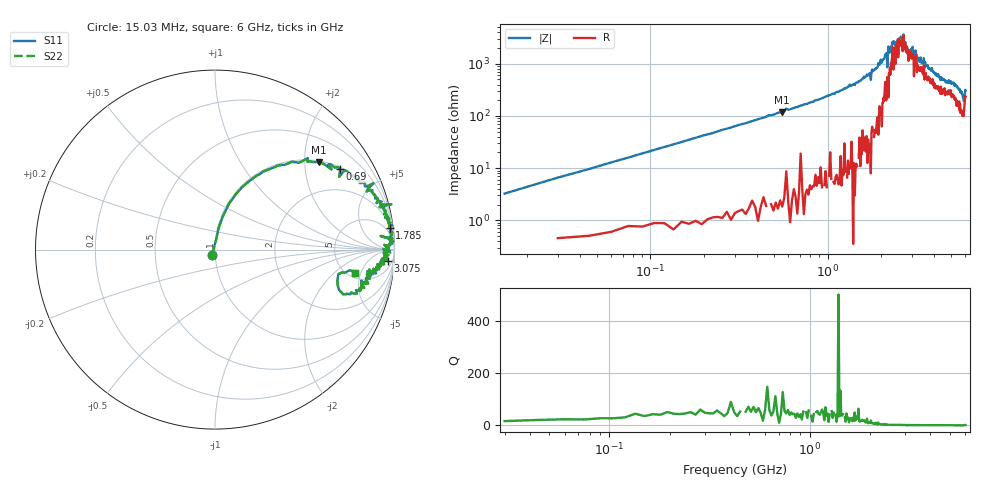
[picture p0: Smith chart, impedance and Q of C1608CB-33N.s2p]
!	Network	Analyzer	HP8753E.07.74:	Oct	30	2002	Serial	No.	JP38451487
!	Hewlett-Packard
!	7	Sep	2009	9:43:19
!	Frequency	S11	S21	S12	S22
#	HZ	S	RI	R	50
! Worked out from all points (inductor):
!   400 points, 15.03 MHz to 6 GHz, reference 50 ohm
!   read as one part in series: L = 33.9 nH near 45.03 MHz
!   highest Q = 58.1 at 555 MHz (marker M1), where L = 33.7 nH
!   self-resonance near 2.53 GHz
!   S11 on the Smith chart (normalised r, x): 15.03 MHz: 0.97, -0.05; 690 MHz: 1.07, +3.07; 1.785 GHz: 2, +16; 3.075 GHz: 12, -24; 6 GHz: 5.75, -3.94
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1.502992e7  -0.0166 -0.0276  1.02 0.0276  1.02 0.0276  -0.0166 -0.0276
6.00297e7  0.0219 0.125  0.978 -0.125  0.978 -0.125  0.0219 0.125
1.650292e8  0.115 0.307  0.885 -0.307  0.885 -0.307  0.115 0.307
5.550272e8  0.579 0.486  0.421 -0.486  0.421 -0.486  0.579 0.486
6.900266e8  0.698 0.448  0.302 -0.448  0.302 -0.448  0.698 0.448
1.020025e9  0.853 0.34  0.147 -0.34  0.147 -0.34  0.853 0.34
1.785021e9  0.974 0.123  0.0256 -0.123  0.0256 -0.123  0.974 0.123
2.01002e9  0.981 0.0887  0.0186 -0.0887  0.0186 -0.0887  0.981 0.0887
2.145019e9  0.988 0.0611  0.0116 -0.0611  0.0116 -0.0611  0.988 0.0611
2.175019e9  0.923 0.076  0.0769 -0.076  0.0769 -0.076  0.923 0.076
2.205019e9  0.993 0.0458  0.00702 -0.0458  0.00702 -0.0458  0.993 0.0458
2.325018e9  0.97 0.0213  0.0303 -0.0213  0.0303 -0.0213  0.97 0.0213
2.505017e9  0.943 0.0267  0.0573 -0.0267  0.0573 -0.0267  0.943 0.0267
2.595017e9  0.976 -0.0163  0.0245 0.0163  0.0245 0.0163  0.976 -0.0163
2.655017e9  0.95 -0.0153  0.0496 0.0153  0.0496 0.0153  0.95 -0.0153
2.685017e9  0.974 -0.00583  0.0261 0.00583  0.0261 0.00583  0.974 -0.00583
2.865016e9  0.946 -0.0382  0.0535 0.0382  0.0535 0.0382  0.946 -0.0382
3.015015e9  0.966 -0.0301  0.0344 0.0301  0.0344 0.0301  0.966 -0.0301
3.075015e9  0.964 -0.0637  0.0364 0.0637  0.0364 0.0637  0.964 -0.0637
4.00501e9  0.915 -0.109  0.0853 0.109  0.0853 0.109  0.915 -0.109
5.010005e9  0.857 -0.138  0.143 0.138  0.143 0.138  0.857 -0.138
6e9  0.779 -0.129  0.221 0.129  0.221 0.129  0.779 -0.129
